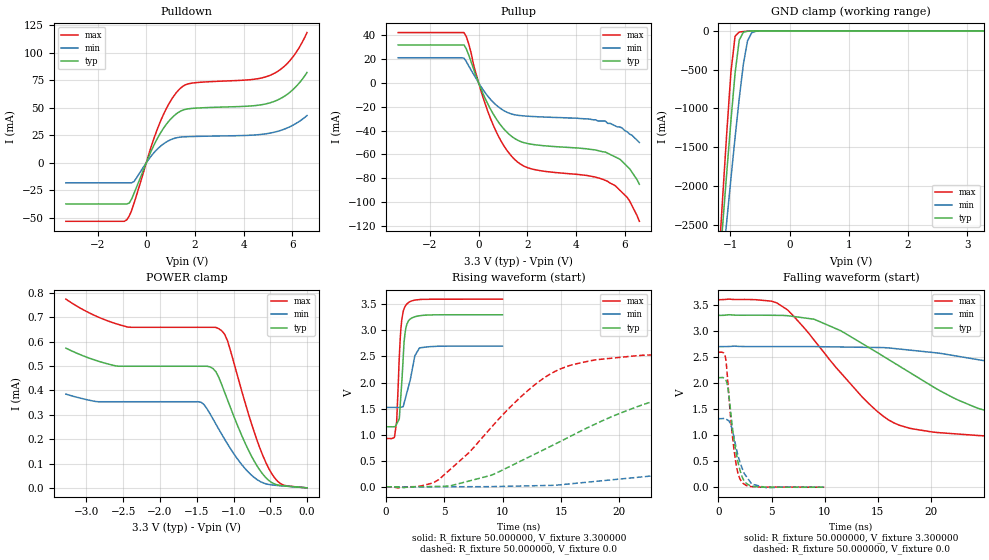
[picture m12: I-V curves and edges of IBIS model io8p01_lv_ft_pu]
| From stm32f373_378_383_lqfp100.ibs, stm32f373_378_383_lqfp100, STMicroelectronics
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|   Model io8p01_lv_ft_pu
[Model]  io8p01_lv_ft_pu
Model_type I/O
Polarity   Non-Inverting
Enable   Active-Low
Vinl =   0.990000V
Vinh =   2.310000V
Vmeas =  1.650000V
Cref =   50.000000pF
Rref =   100.000000M
Vref =   0.0V
C_comp   5.028100pF   4.857200pF   5.254400pF
[Temperature Range]   25.000000   0.125000k   -40.000000
[Pullup Reference]   3.300000V   2.700000V   3.600000V
[Pulldown Reference]   0.0V   0.0V   0.0V
[POWER Clamp Reference]   3.300000V   2.700000V   3.600000V
[GND Clamp Reference]   0.0V   0.0V   0.0V
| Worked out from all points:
|   slope of the pulldown table from 0 to 0.495 V, typ, clamps not added: 20.9 ohm
|   slope of the pullup table from 0 to 0.495 V, typ, clamps not added: 22.2 ohm
|   GND clamp passes 1 mA (typ) near -0.59 V on its own axis
|   rising waveform, R_fixture 50.000000, V_fixture 3.300000: 20-80 % time 371ps typ, 696ps min, 337ps max; typ from 1.15 V to 3.3 V
|   rising waveform, R_fixture 50.000000, V_fixture 0.0: 20-80 % time 12.6ns typ, 30.6ns min, 7.02ns max; typ from 0.001 V to 2.1 V
|   falling waveform, R_fixture 50.000000, V_fixture 3.300000: 20-80 % time 11ns typ, 22.7ns min, 6.89ns max; typ from 3.3 V to 1.15 V
|   falling waveform, R_fixture 50.000000, V_fixture 0.0: 20-80 % time 883ps typ, 1.07ns min, 740ps max; typ from 2.1 V to 0.001 V
[Pulldown]
|Voltage   I(typ)   I(min)   I(max)
-3.3V     -37.45mA   -18.2mA    -53.24mA
-800mV    -37.45mA   -18.2mA    -51.9mA
-700mV    -36.7mA    -18.2mA    -48.48mA
-500mV    -27.71mA   -17.01mA   -36.66mA
500mV     23.91mA    13.38mA    33.24mA
900mV     37.17mA    19.88mA    52.48mA
1.3V      45.55mA    23.01mA    65.5mA
1.8V      49.29mA    23.83mA    72.18mA
4.4V      51.88mA    25.21mA    75.91mA
5.2V      55.41mA    27.53mA    80.72mA
5.9V      64.2mA     32.82mA    93.01mA
6.6V      82.13mA    42.97mA    118.5mA
[Pullup]
|Voltage   I(typ)   I(min)   I(max)
-3.3V     31.7mA     20.96mA    42.04mA
-600mV    31.7mA     20.58mA    42.04mA
-400mV    22.99mA    13.87mA    32.11mA
0V        100fA      16.1pA     0A
500mV     -22.5mA    -14.16mA   -30.52mA
900mV     -35.28mA   -21.54mA   -48mA
1.4V      -45.54mA   -26.4mA    -62.54mA
2.2V      -51.57mA   -28.22mA   -72.25mA
4.5V      -55.5mA    -30.3mA    -77.84mA
5.3V      -59mA      -34mA      -82.6mA
6.1V      -70mA      -41mA      -96mA
6.6V      -85mA      -50mA      -116mA
[GND_clamp]
|Voltage   I(typ)   I(min)   I(max)
-3.3V     -9.706A    -9.438A    -9.292A
-1.2V     -3.211A    -3.571A    -3.02A
-1.13V    -2.511A    -3.008A    -2.153A
-1.06V    -1.824A    -2.453A    -1.311A
-990mV    -1.16A     -1.907A    -534mA
-920mV    -548mA     -1.377A    -70.08mA
-850mV    -120.4mA   -875.9mA   -15.9mA
-780mV    -17.66mA   -430.9mA   -9.191mA
-710mV    -5.44mA    -130.8mA   -5.02mA
-640mV    -2.077mA   -25.65mA   -2.003mA
-570mV    -540.4uA   -6.293mA   -433.9uA
3.28V     0A         0A         0A
[POWER_clamp]
|Voltage   I(typ)   I(min)   I(max)
-3.28V    574uA      385.1uA    775.2uA
-2.88V    524.3uA    354.9uA    706.9uA
-2.44V    499.5uA    353.8uA    660.7uA
-1.44V    499.5uA    351.5uA    659.5uA
-1.28V    490.2uA    283.5uA    659.5uA
-1.16V    423.6uA    220uA      645.1uA
-1.08V    360.3uA    179.6uA    602.6uA
-800mV    157uA      65.19uA    307.1uA
-640mV    71.83uA    26.56uA    162.4uA
-520mV    30.52uA    13.8uA     79.51uA
-360mV    9.626uA    8.662uA    17.31uA
0V        0A         0A         0A
[Ramp]
| variable   typ   min   max
dV/dt_r  1.26198/12.63093n   0.78958/30.60141n   1.55427/7.01265n
dV/dt_f  1.28874/11.01884n   0.70632/22.77902n   1.60395/6.88266n
R_load = 50.000000
[Rising Waveform]
R_fixture= 50.000000
V_fixture= 3.300000
V_fixture_min= 2.700000
V_fixture_max= 3.600000
|time   V(typ)   V(min)   V(max)
0s        1.152V     1.524V     926.8mV
720.7ps   1.154V     1.523V     966.6mV
900.9ps   1.206V     1.522V     1.255V
1.121ns   1.302V     1.524V     2.458V
1.341ns   2.013V     1.531V     3.205V
1.542ns   2.789V     1.608V     3.419V
1.742ns   3.091V     1.776V     3.499V
2.462ns   3.262V     2.515V     3.582V
2.863ns   3.281V     2.666V     3.592V
9.97ns    3.3V       2.7V       3.6V
[Rising Waveform]
R_fixture= 50.000000
V_fixture= 0.0
V_fixture_min= 0.0
V_fixture_max= 0.0
|time   V(typ)   V(min)   V(max)
0s        1.1mV      1.225mV    1.052mV
4.505ns   8.884mV    3.013mV    137.1mV
9.009ns   222.5mV    4.75mV     1.139V
14.51ns   822.9mV    30.43mV    2.218V
22.02ns   1.576V     192.9mV    2.524V
28.53ns   1.911V     356.9mV    2.57V
38.54ns   2.054V     653.9mV    2.589V
57.56ns   2.098V     1.08V      2.592V
78.58ns   2.105V     1.256V     2.592V
249.2ns   2.104V     1.317V     2.592V
[Falling Waveform]
R_fixture= 50.000000
V_fixture= 3.300000
V_fixture_min= 2.700000
V_fixture_max= 3.600000
|time   V(typ)   V(min)   V(max)
0s        3.3V       2.7V       3.6V
5.005ns   3.302V     2.701V     3.572V
6.507ns   3.294V     2.701V     3.405V
11.51ns   3.005V     2.693V     2.199V
16.52ns   2.391V     2.665V     1.237V
25.03ns   1.482V     2.43V      987.8mV
33.03ns   1.273V     2.139V     948.6mV
46.05ns   1.191V     1.765V     931.9mV
74.07ns   1.155V     1.573V     926.9mV
249.2ns   1.152V     1.524V     926.8mV
[Falling Waveform]
R_fixture= 50.000000
V_fixture= 0.0
V_fixture_min= 0.0
V_fixture_max= 0.0
|time   V(typ)   V(min)   V(max)
0s        2.104V     1.317V     2.592V
660.7ps   2.07V      1.317V     2.488V
900.9ps   1.888V     1.284V     1.967V
1.221ns   1.313V     1.161V     1.166V
1.522ns   832.7mV    895.4mV    631.2mV
1.862ns   463.7mV    590.7mV    249.6mV
2.282ns   174.9mV    337.8mV    82.85mV
3.123ns   25.44mV    63.81mV    12.73mV
4.565ns   2.602mV    -10.29mV   4.5mV
9.97ns    1.1mV      1.225mV    1.052mV
